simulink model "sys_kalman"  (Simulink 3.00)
settings: Solver=ode45  StartTime=0.0  StopTime=Tstop  MaxStep=max_step  RelTol=1e-3
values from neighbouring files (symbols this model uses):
  den = [0.02 1]    [lsg_regelung_ini.m]    (also in lsg_system_ini.m; lsg_sys_kalman_ini.m; system_ini.m; sys_kalman_ini.m)
  g = 2    [lsg_regelung_ini.m]    (also in lsg_system_ini.m; lsg_sys_kalman_ini.m; system_ini.m; sys_kalman_ini.m)
  num = 2    [lsg_regelung_ini.m]    (also in lsg_system_ini.m; lsg_sys_kalman_ini.m; system_ini.m; sys_kalman_ini.m)
  p = [-2 -3+10*i -3-10*i]    [lsg_regelung_ini.m]    (also in lsg_system_ini.m; lsg_sys_kalman_ini.m; system_ini.m; sys_kalman_ini.m)
  Q = 1e-3    (= 0.001)    [lsg_regelung_ini.m]    (also in lsg_sys_kalman_ini.m; sys_kalman_ini.m = 1e-06)
  R = 1e-3    (= 0.001)    [lsg_regelung_ini.m]    (also in lsg_sys_kalman_ini.m; sys_kalman_ini.m = 1e-06)
  verst = 100    [lsg_regelung_ini.m]    (also in lsg_system_ini.m; lsg_sys_kalman_ini.m; system_ini.m; sys_kalman_ini.m)
  z = [1 1]    [lsg_regelung_ini.m]    (also in lsg_system_ini.m; lsg_sys_kalman_ini.m; system_ini.m; sys_kalman_ini.m)

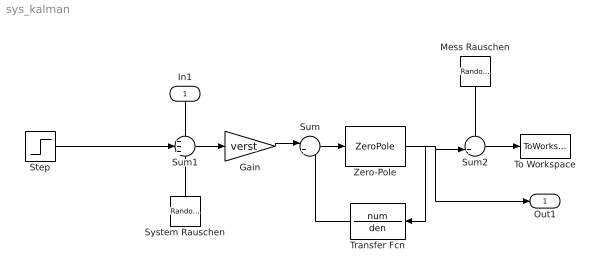
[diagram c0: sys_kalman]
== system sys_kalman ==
  In1 : Inport  Orientation=down  Port=1  PortWidth=-1  SampleTime=-1  DataType=auto
  Gain : Gain  Gain=verst  SaturateOnIntegerOverflow=on
  Mess Rauschen : RandomNumber  Orientation=down  Mean=0  Variance=R  Seed=0  SampleTime=0
  Step : Step  Time=1  Before=0  After=1  SampleTime=0
  Sum : Sum  Inputs=|++  SaturateOnIntegerOverflow=on
  Sum1 : Sum  Inputs=+++  SaturateOnIntegerOverflow=on
  Sum2 : Sum  Inputs=++|  SaturateOnIntegerOverflow=on
  System Rauschen : RandomNumber  Orientation=up  Mean=0  Variance=Q  Seed=0  SampleTime=0
  To Workspace : ToWorkspace  VariableName=y  SampleTime=-1  SaveFormat=Matrix
  Transfer Fcn : TransferFcn  Orientation=left  Numerator=num  Denominator=den
  Zero-Pole : ZeroPole  Zeros=z  Poles=p  Gain=g
  Out1 : Outport  Port=1
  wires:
  Transfer Fcn/1 -> Sum/2
  Sum/1 -> Zero-Pole/1
  Gain/1 -> Sum/1
  Zero-Pole/1 -> Transfer Fcn/1, Sum2/2, Out1/1
  Mess Rauschen/1 -> Sum2/1
  In1/1 -> Sum1/1
  System Rauschen/1 -> Sum1/3
  Sum1/1 -> Gain/1
  Step/1 -> Sum1/2
  Sum2/1 -> To Workspace/1
